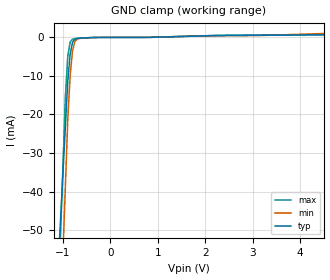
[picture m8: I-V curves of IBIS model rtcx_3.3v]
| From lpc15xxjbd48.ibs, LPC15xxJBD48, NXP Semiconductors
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[Model] rtcx_3.3v
Model_type Input
Vinl = 990.000mV
Vinh = 2.31000V
C_comp 1.24000pF 1.24000pF 1.24000pF
| variable typ   min   max
[Voltage Range] 3.30000V 3.00000V 3.60000V
[POWER Clamp Reference] 3.30000V 3.00000V 3.60000V
[GND Clamp Reference] 0.00000V 0.00000V 0.00000V
[Temperature Range]   25   85   -40
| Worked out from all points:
|   GND clamp passes 1 mA (typ) near -0.78 V on its own axis
[GND Clamp]
-3.3V     -577.6mA   -843mA     -835.5mA
-950mV    -23.25mA   -38.59mA   -15.43mA
-900mV    -11.45mA   -21.48mA   -4.949mA
-850mV    -4.408mA   -10.01mA   -1.212mA
-800mV    -1.3mA     -3.528mA   -464.7uA
-750mV    -465.7uA   -1.067mA   -342uA
-700mV    -265.9uA   -414.5uA   -219.3uA
-600mV    -162.8uA   -156.4uA   -160uA
3.2V      559.9uA    502.9uA    615uA
6.6V      836.7uA    1.839mA    900.6uA
[POWER Clamp]
-3.3V     0A         0A         0A
6.6V      0A         0A         0A
